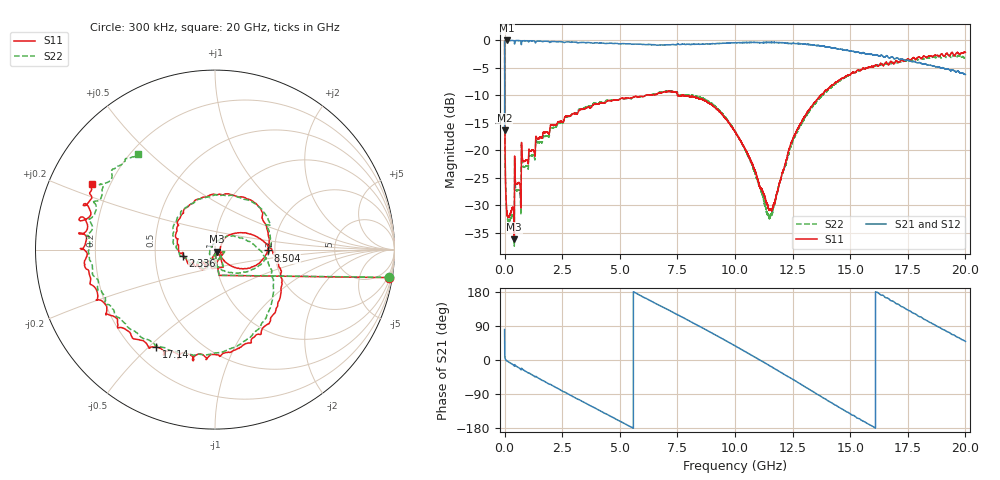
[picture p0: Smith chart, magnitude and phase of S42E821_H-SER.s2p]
!{S42E821}
!Johanson Technology Inc.
!www.johansontechnology.com
!Test Board Conditions:
!Substrate Type  RO4350B
!Substrate Thickness  50 mil
!Substrate Dk  3.66
!TL Type: GCPW
!TL Trace Width  60 mil
!TL Gap  10 mil
!Electrode orientation  Horizontal
!DUT TOPOLOGY	SERIES
!Mounting Pad LxW  14x55 mil
! Created Wed Nov 25 22:28:03 2020
# khz S ma R 50
! 2 Port Network Data from SP1.SP block
! freq  magS11  angS11  magS21  angS21  magS12  angS12  magS22  angS22
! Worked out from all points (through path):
!   20001 points, 300 kHz to 20 GHz, reference 50 ohm
!   highest |S21| = -0.03 dB at 102.3 MHz (marker M1); lowest = -16.4 dB at 300 kHz (marker M2)
!   group delay of S21, straight-line fit = 93.8 ps
!   lowest |S11| = -36.2 dB at 421.3 MHz (marker M3), VSWR 1.03, Z = 51 - j1.22 ohm
!   |S11| at or under -10 dB: 5.86 MHz to 6.124 GHz (6.118 GHz wide, 200 % of centre); 7.5 GHz to 7.719 GHz (219 MHz wide, 2.88 % of centre); 7.766 GHz to 13.72 GHz (5.949 GHz wide, 55.4 % of centre)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
!   |S22| runs from -37.4 to -0.1 dB; largest |S21 - S12| = 0.017
!   S11 on the Smith chart (normalised r, x): 300 kHz: 1, -12; 2.336 GHz: 0.70, -0.05; 8.504 GHz: 1.83, -0.02; 17.14 GHz: 0.29, -0.53; 20 GHz: 0.13, +0.25
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300  0.9819 -9.1  0.152 80.5  0.1514 80.4  0.9837 -9.0
102300  0.02697 -84.4  0.9963 -2.3  0.9948 -2.4  0.02595 -84.2
202300  0.02512 -89.1  0.9957 -6.2  0.9952 -6.2  0.02232 -89.2
421300  0.01547 -50.6  0.9851 -15.5  0.9852 -15.4  0.01422 -33.4
820300  0.07899 -114.9  0.9899 -26.5  0.9899 -26.5  0.0704 -115.4
2336300  0.1818 -168.4  0.9704 -76.0  0.9704 -76.0  0.1754 -166.5
3334300  0.2355 157.1  0.9564 -108.0  0.9561 -108.0  0.2388 166.2
5139300  0.2963 108.5  0.9322 -165.6  0.9318 -165.5  0.2943 105.6
6667300  0.33 62.9  0.9037 146.0  0.9026 145.9  0.3342 55.0
7599300  0.3129 30.8  0.915 116.7  0.9171 116.6  0.3137 23.4
8504300  0.2933 -0.9  0.9205 87.2  0.9192 87.4  0.3013 -2.6
1.00003e7  0.1484 -42.4  0.949 37.4  0.9479 37.4  0.1495 -58.5
1.08063e7  0.07022 -51.3  0.9556 9.4  0.9556 9.3  0.06676 -105.1
1.15253e7  0.02888 -5.6  0.9557 -15.8  0.9562 -15.8  0.0249 144.7
1.24863e7  0.1232 43.6  0.9359 -50.2  0.9358 -50.3  0.116 40.2
1.33343e7  0.2515 14.7  0.9102 -81.7  0.9096 -81.7  0.2438 0.5
1.40713e7  0.3663 -14.4  0.8692 -109.0  0.8711 -108.6  0.3604 -26.7
1.50253e7  0.4933 -51.1  0.7943 -143.1  0.798 -143.2  0.4883 -58.0
1.66673e7  0.6002 -105.2  0.6969 161.9  0.6991 161.0  0.6158 -113.1
1.71373e7  0.6359 -121.1  0.6696 144.9  0.6736 144.1  0.6382 -129.7
1.88053e7  0.726 -175.3  0.5736 87.8  0.5702 88.2  0.7068 174.2
2e7  0.7751 152.0  0.4885 49.2  0.4892 49.6  0.6872 128.6
